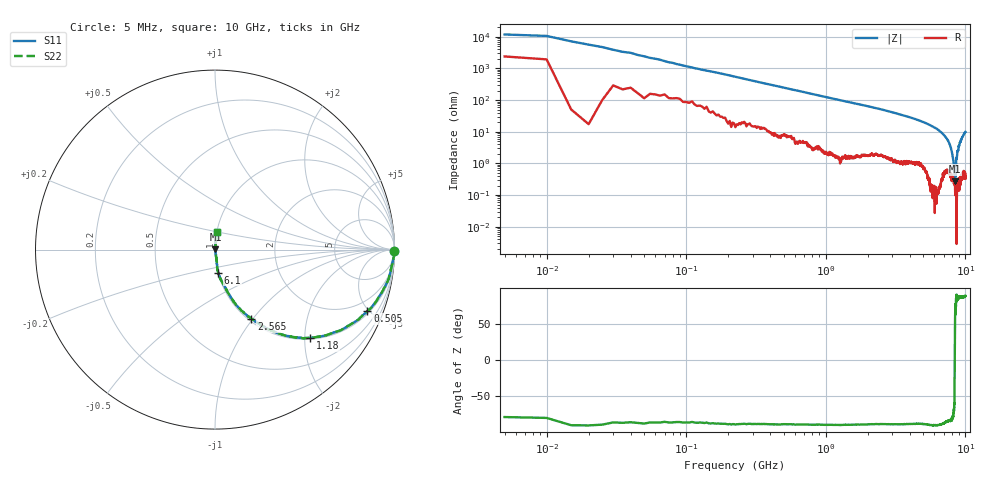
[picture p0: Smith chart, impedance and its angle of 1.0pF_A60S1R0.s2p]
! Amotech Co.,Ltd.
! http://www.amotech.co.kr/
! Part Number: A60S1R0
! These Parameters are Measured in Series Mode Connection
! Operation Temp=25[degC], DC Bias Voltage=0[V]
! Freq. Start=5[MHz] Stop=10[GHz], 2000[Steps]
! Date: Monday, July 13, 2020, 01:24:45
# GHZ S RI R 50.000000
!Freq.(Hz) S11(Real) S11(Imag) S21(Real) S21(Imag) S12(Real) S12(Imag) S22(Real) S22(Imag)
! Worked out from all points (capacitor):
!   2000 points, 5 MHz to 10 GHz, reference 50 ohm
!   read as one part in series: C = 1.36 pF near 55 MHz
!   lowest |Z| = 270 mohm at 8.415 GHz (marker M1)
!   series resonance near 8.398 GHz, so ESL is about 260 pH
!   S11 on the Smith chart (normalised r, x): 5 MHz: open; 505 MHz: 1.15, -4.90; 1.18 GHz: 1.03, -2.12; 2.565 GHz: 1.03, -0.98; 6.1 GHz: 1.00, -0.26; 10 GHz: 1.01, +0.20
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0.005  0.9982 -0.00827  0.00178 0.00827  0.00178 0.00827  0.9982 -0.00827
0.08  0.9906 -0.0657  0.00938 0.0657  0.00938 0.0657  0.9906 -0.0657
0.15  0.9789 -0.1209  0.0211 0.1209  0.0211 0.1209  0.9789 -0.1209
0.295  0.938 -0.2239  0.062 0.2239  0.062 0.2239  0.938 -0.2239
0.505  0.8495 -0.3424  0.1505 0.3424  0.1505 0.3424  0.8495 -0.3424
1.18  0.5287 -0.4911  0.4713 0.4911  0.4713 0.4911  0.5287 -0.4911
1.675  0.3671 -0.471  0.6329 0.471  0.6329 0.471  0.3671 -0.471
2.565  0.2029 -0.3857  0.7971 0.3857  0.7971 0.3857  0.2029 -0.3857
3.34  0.1208 -0.3113  0.8792 0.3113  0.8792 0.3113  0.1208 -0.3113
5.005  0.0446 -0.19  0.9554 0.19  0.9554 0.19  0.0446 -0.19
6.1  0.0182 -0.1278  0.9818 0.1278  0.9818 0.1278  0.0182 -0.1278
6.67  0.0119 -0.0971  0.9881 0.0971  0.9881 0.0971  0.0119 -0.0971
7.38  0.00948 -0.0585  0.9905 0.0585  0.9905 0.0585  0.00948 -0.0585
7.835  0.00514 -0.0329  0.9949 0.0329  0.9949 0.0329  0.00514 -0.0329
8.175  0.00307 -0.0131  0.9969 0.0131  0.9969 0.0131  0.00307 -0.0131
8.335  0.00217 -0.00405  0.9978 0.00405  0.9978 0.00405  0.00217 -0.00405
8.415  0.00228 0.00143  0.9977 -0.00143  0.9977 -0.00143  0.00228 0.00143
8.465  0.00112 0.00425  0.9989 -0.00425  0.9989 -0.00425  0.00112 0.00425
8.595  0.00177 0.0122  0.9982 -0.0122  0.9982 -0.0122  0.00177 0.0122
8.795  0.00225 0.0243  0.9977 -0.0243  0.9977 -0.0243  0.00225 0.0243
9.155  0.00499 0.0445  0.995 -0.0445  0.995 -0.0445  0.00499 0.0445
10  0.0131 0.098  0.9869 -0.098  0.9869 -0.098  0.0131 0.098
